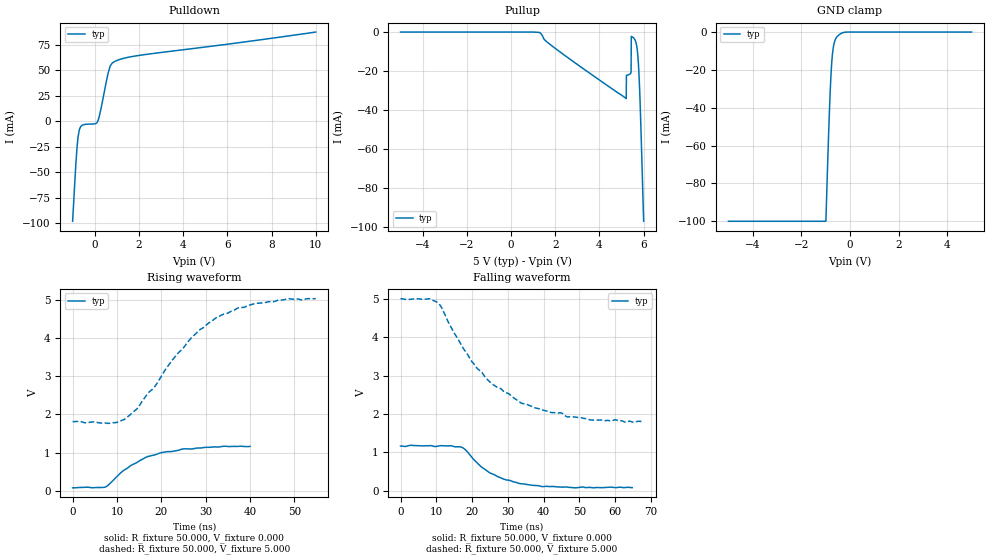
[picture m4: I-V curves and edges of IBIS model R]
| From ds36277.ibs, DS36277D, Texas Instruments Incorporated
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|   Model R
[Model]   R
Model_type   3-state
Vmeas = 2.5
|   typ   min   max
|   (nom PVT)   (fast PVT)   (slow PVT)
C_comp   6.336pF   NA   NA
[Voltage Range]   5   NA   NA
[Temperature Range]   27   NA   NA
[Power Clamp Reference]   5   NA   NA
[GND Clamp Reference]   0   0   0
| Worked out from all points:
|   slope of the pulldown table from 0 to 0.75 V, typ, clamps not added: 12.9 ohm
|   GND clamp passes 1 mA (typ) near -0.40 V on its own axis
|   falling waveform, R_fixture 50.000, V_fixture 0.000: 20-80 % time 9.73ns typ, NA min, NA max; typ from 1.17 V to 0.082 V
|   falling waveform, R_fixture 50.000, V_fixture 5.000: 20-80 % time 17.8ns typ, NA min, NA max; typ from 5 V to 1.8 V
|   rising waveform, R_fixture 50.000, V_fixture 0.000: 20-80 % time 9.34ns typ, NA min, NA max; typ from 0.082 V to 1.17 V
|   rising waveform, R_fixture 50.000, V_fixture 5.000: 20-80 % time 14.2ns typ, NA min, NA max; typ from 1.81 V to 5.03 V
[GND Clamp]
|   Voltage   I(typ)   I(min)  I(max)
-5V       -100mA     NA         NA
-992.1mV  -99.9mA    NA         NA
-911.2mV  -66.23mA   NA         NA
-843.8mV  -40.85mA   NA         NA
-789.9mV  -24.55mA   NA         NA
-749.4mV  -15.79mA   NA         NA
-695.5mV  -8.835mA   NA         NA
-641.6mV  -5.352mA   NA         NA
-574.2mV  -3.215mA   NA         NA
-452.8mV  -1.49mA    NA         NA
-102.2mV  -11.68uA   NA         NA
5V        0A         NA         NA
[Pulldown]
|   Voltage   I(typ)   I(min)   I(max)
-1V       -97.84mA   NA         NA
-850mV    -40.68mA   NA         NA
-800mV    -25.38mA   NA         NA
-750mV    -14.75mA   NA         NA
-700mV    -8.799mA   NA         NA
-540mV    -3.529mA   NA         NA
120mV     -559.6uA   NA         NA
300mV     13.98mA    NA         NA
600mV     46.65mA    NA         NA
800mV     57.28mA    NA         NA
2V        64.56mA    NA         NA
10V       87.47mA    NA         NA
[Pullup]
|   Voltage   I(typ)   I(min)   I(max)
-5V       930nA      NA         NA
1.3V      -227.6uA   NA         NA
1.8V      -6.649mA   NA         NA
5.21V     -34.08mA   NA         NA
5.22V     -22.19mA   NA         NA
5.43V     -20.6mA    NA         NA
5.44V     -2.187mA   NA         NA
5.55V     -3.002mA   NA         NA
5.7V      -8.281mA   NA         NA
5.78V     -19.9mA    NA         NA
5.86V     -43.51mA   NA         NA
6V        -97.04mA   NA         NA
[Ramp]
R_load = 50
|   typ   min   max
dV/dt_r   0.6558/8.82e-9   NA   NA
dV/dt_f   1.908/16.92e-9   NA   NA
[Falling Waveform]
R_fixture = 50.000
V_fixture = 0.000
C_fixture = 0.000
|  time   V(typ)   V(min)   V(max)
0s        1.165V     NA         NA
16.8ns    1.143V     NA         NA
18ns      1.081V     NA         NA
22ns      674.3mV    NA         NA
24.8ns    477.8mV    NA         NA
28.8ns    305.5mV    NA         NA
33.2ns    190.7mV    NA         NA
39.6ns    109mV      NA         NA
48.8ns    77.1mV     NA         NA
64.8ns    82.19mV    NA         NA
[Falling Waveform]
R_fixture = 50.000
V_fixture = 5.000
C_fixture = 0.000
|  time   V(typ)   V(min)   V(max)
0s        5V         NA         NA
8ns       5.003V     NA         NA
10.4ns    4.897V     NA         NA
17.2ns    3.762V     NA         NA
21.2ns    3.214V     NA         NA
25.6ns    2.782V     NA         NA
34ns      2.275V     NA         NA
44.8ns    2.033V     NA         NA
46.8ns    1.922V     NA         NA
68ns      1.805V     NA         NA
[Rising Waveform]
R_fixture = 50.000
V_fixture = 0.000
C_fixture = 0.000
|  time   V(typ)   V(min)   V(max)
0s        82.19mV    NA         NA
7.6ns     114.3mV    NA         NA
11.2ns    511.4mV    NA         NA
13.2ns    670.8mV    NA         NA
16.8ns    894.4mV    NA         NA
20ns      1.002V     NA         NA
24.8ns    1.097V     NA         NA
30ns      1.141V     NA         NA
34ns      1.169V     NA         NA
40ns      1.165V     NA         NA
[Rising Waveform]
R_fixture = 50.000
V_fixture = 5.000
C_fixture = 0.000
|  time   V(typ)   V(min)   V(max)
0s        1.812V     NA         NA
8.4ns     1.769V     NA         NA
12ns      1.9V       NA         NA
14.8ns    2.185V     NA         NA
22.4ns    3.409V     NA         NA
26.4ns    3.956V     NA         NA
32.8ns    4.553V     NA         NA
41.2ns    4.902V     NA         NA
48.4ns    5.025V     NA         NA
54.8ns    5.028V     NA         NA
